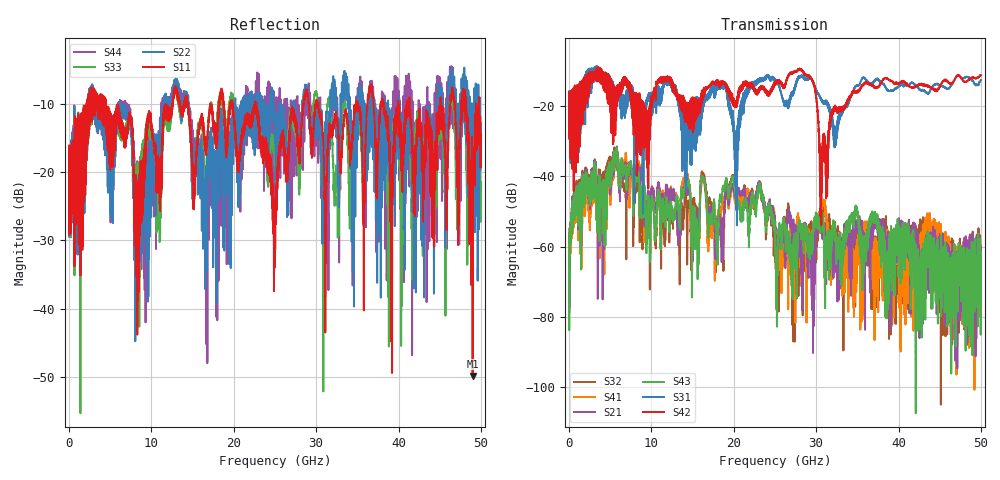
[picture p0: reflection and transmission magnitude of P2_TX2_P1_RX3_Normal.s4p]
!Keysight Technologies,N5225B,MY57041031,A.13.20.10
!Date: Friday, May 31, 2019 11:18:06
!Correction: S11(Full 4 Port(1,2,3,4))
!S12(Full 4 Port(1,2,3,4))
!S13(Full 4 Port(1,2,3,4))
!S14(Full 4 Port(1,2,3,4))
!S21(Full 4 Port(1,2,3,4))
!S22(Full 4 Port(1,2,3,4))
!S23(Full 4 Port(1,2,3,4))
!S24(Full 4 Port(1,2,3,4))
!S31(Full 4 Port(1,2,3,4))
!S32(Full 4 Port(1,2,3,4))
!S33(Full 4 Port(1,2,3,4))
!S34(Full 4 Port(1,2,3,4))
!S41(Full 4 Port(1,2,3,4))
!S42(Full 4 Port(1,2,3,4))
!S43(Full 4 Port(1,2,3,4))
!S44(Full 4 Port(1,2,3,4))
!S4P File: Measurements: <S11,S12,S13,S14>,
!<S21,S22,S23,S24>,
!<S31,S32,S33,S34>,
!<S41,S42,S43,S44>:
# Hz S  dB  R 50.0
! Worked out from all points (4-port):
!   5000 points, 10 MHz to 50 GHz, reference 50 ohm
!   strongest paths, dB at 10 MHz, 12.51 GHz, 25.01 GHz, 37.51 GHz, 50 GHz:
!     S42: -19.7, -14.4, -13.2, -14.5, -11.2
!     S31: -19.3, -14.9, -13.0, -12.4, -12.6
!     S43: -56.2, -49.5, -59.1, -54.3, -64.4
!     S21: -61.4, -46.8, -53.4, -55.3, -65.3
!     S41: -54.9, -46.2, -56.1, -63.8, -65.4
!     S32: -58.8, -52.7, -63.4, -63.0, -70.5
!   lowest |S11| = -49.9 dB at 49 GHz (marker M1), VSWR 1.01, Z = 49.7 + j0.0679 ohm
!   |S11| at or under -10 dB: 4.481 GHz to 11.72 GHz (7.238 GHz wide, 89.4 % of centre); 22.73 GHz to 28.47 GHz (5.744 GHz wide, 22.4 % of centre); 30.26 GHz to 34.82 GHz (4.562 GHz wide, 14 % of centre)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
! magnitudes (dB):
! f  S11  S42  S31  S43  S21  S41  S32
! 10 MHz  -19.2  -19.7  -19.3  -56.2  -61.4  -54.9  -58.8
! 5.67 GHz  -14.4  -24.1  -17.1  -33.1  -33.2  -33.7  -32.4
! 20.24 GHz  -14.5  -20.2  -32.3  -46.5  -45.5  -47.0  -44.6
! 28.07 GHz  -15.3  -9.3  -11.5  -55.8  -63.1  -59.4  -58.6
! 30.63 GHz  -12.3  -40.6  -18.4  -52.5  -56.3  -49.8  -51.3
! 49 GHz  -49.9  -11.8  -12.7  -60.6  -68.6  -66.1  -58.0
! 50 GHz  -14.4  -11.2  -12.6  -64.4  -65.3  -65.4  -70.5
